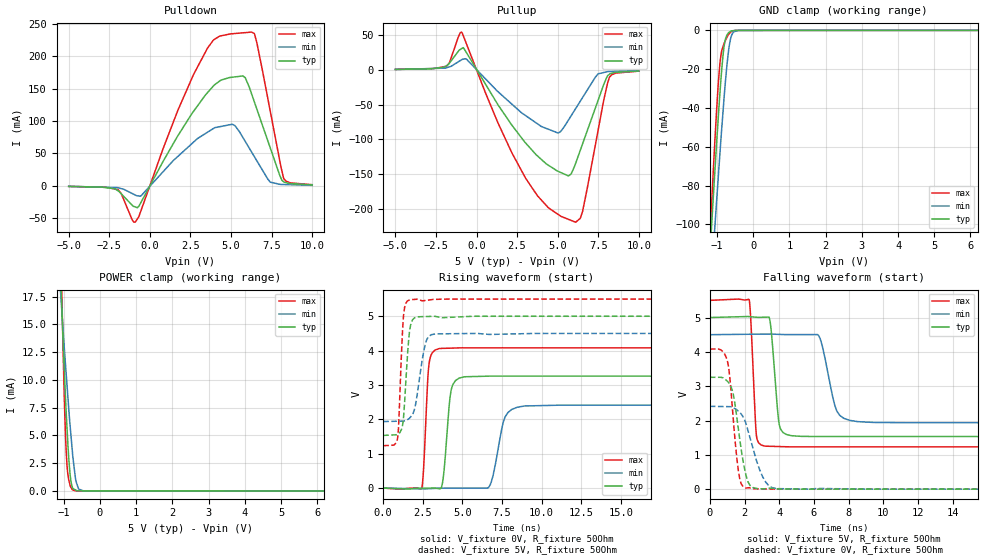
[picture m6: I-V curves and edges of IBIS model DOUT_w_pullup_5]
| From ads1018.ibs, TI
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|   DOUT Model 5 V model  Config Register bit3=0
[Model] DOUT_w_pullup_5
|  Signals  DOUT/_DRDY(9)
|   bit 3 of the Config Registor is zero
Model_type   3-state
Polarity   Non-Inverting
Enable   Active-Low
Vmeas = 2.5
Vref = 2.5
Cref = 15pF
Rref = 50|
|   typ   min   max
|   (nom PVT)   (Fast PVT)   (slow PVT)
C_comp   1.8834020e-12  1.5236910e-12  2.2665370e-12
|   typ   min   max
|   (nom PVT)   (slow PVT)   (Fast PVT)
|C_comp (ON state)   2.6065280e-12  2.2751560e-12  4.1907400e-12
|C_comp (OFF state)   2.4127670e-12  2.2979320e-12  3.1339800e-12
| Where   nom PVT is  Nominal Process, 5V, 27C
|   Fast PVT is Strong or Fast Process, 5.5V, -40C
|   Slow PVT is Weak or Slow Process, 4.5V, 125C
| variable   typ   min   max
[Voltage Range]   5   4.5   5.5
[Temperature Range]   27   125   -40
|Operating Temperature   27   125   -40
[Pullup Reference]   5   4.5   5.5
[Pulldown Reference]   0   0   0
[Power Clamp Reference]   5   4.5   5.5
[GND Clamp Reference]   0   0   0
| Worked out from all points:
|   slope of the pulldown table from 0 to 0.75 V, typ, clamps not added: 21.6 ohm
|   slope of the pullup table from 0 to 0.75 V, typ, clamps not added: 25.9 ohm
|   GND clamp passes 1 mA (typ) near -0.67 V on its own axis
|   POWER clamp passes 1 mA (typ) near -0.81 V on its own axis
|   falling waveform, V_fixture 5V, R_fixture 50Ohm: 20-80 % time 327ps typ, 636ps min, 228ps max; typ from 5 V to 1.53 V
|   rising waveform, V_fixture 0V, R_fixture 50Ohm: 20-80 % time 342ps typ, 600ps min, 247ps max; typ from 0 V to 3.26 V
|   rising waveform, V_fixture 5V, R_fixture 50Ohm: 20-80 % time 296ps typ, 513ps min, 232ps max; typ from 1.53 V to 5 V
|   falling waveform, V_fixture 0V, R_fixture 50Ohm: 20-80 % time 566ps typ, 869ps min, 426ps max; typ from 3.26 V to 0 V
[Pulldown]
|   Voltage   I(typ)   I(min)   I(max)
-5V       -725.3uA   -519.1uA   -702.5uA
-1.982V   -7.151mA   -2.659mA   -5.43mA
-904.6mV  -32.3mA    -13.94mA   -55.69mA
1.743V    78.08mA    45.97mA    117.7mA
3.543V    143.6mA    82.65mA    212mA
5.073V    167.5mA    95.02mA    234.4mA
5.878V    166.7mA    68.46mA    236.2mA
6.262V    142mA      52.38mA    237mA
6.588V    118.4mA    38.77mA    220.8mA
7.411V    58.87mA    5.98mA     115.6mA
8.232V    6.647mA    2.238mA    12.34mA
10V       1.629mA    964.4uA    1.981mA
[GND Clamp]
|   Voltage   I(typ)   I(min)   I(max)
-5V       -1.404A    -1.291A    -1.638A
-1.227V   -124.7mA   -148.3mA   -117.9mA
-1.165V   -105mA     -130.4mA   -94.43mA
-1.148V   -99.65mA   -125.6mA   -88.3mA
-1.058V   -71.83mA   -100.5mA   -56.01mA
-970.8mV  -46.2mA    -76.72mA   -28.63mA
-913.3mV  -30.33mA   -61.39mA   -15.69mA
-788.4mV  -6.224mA   -30.65mA   -6.039mA
-679.5mV  -1.158mA   -10.05mA   -2.032mA
-611.3mV  -337.6uA   -3.284mA   -608uA
-399.6mV  -32.58uA   -25.18uA   -58.78uA
10V       0A         0A         0A
[Pullup]
|   Voltage   I(typ)   I(min)   I(max)
-5V       576.2uA    454.8uA    606.3uA
-1.857V   5.713mA    2.967mA    5.127mA
-922.9mV  30.49mA    14.44mA    54.34mA
1.341V    -51.05mA   -31.91mA   -77.47mA
3.01V     -105.1mA   -65.73mA   -155.5mA
5.031V    -146.2mA   -91mA      -208.3mA
5.667V    -152.8mA   -72.14mA   -215.4mA
6.1V      -134.9mA   -56mA      -219.4mA
6.533V    -106.5mA   -39.85mA   -203.8mA
7.481V    -44.37mA   -5.99mA    -88.03mA
8.171V    -6.695mA   -2.423mA   -11.57mA
10V       -1.583mA   -1.032mA   -1.861mA
[POWER Clamp]
|   Voltage   I(typ)   I(min)   I(max)
-5V       476.7mA    315.9mA    750.7mA
-1.072V   18.22mA    17.1mA     20.63mA
-1.047V   15.95mA    15.84mA    16.68mA
-970.8mV  9.805mA    12.19mA    6.818mA
-944.3mV  7.828mA    11.02mA    4.358mA
-913.3mV  5.861mA    9.651mA    2.434mA
-825.6mV  1.5mA      5.9mA      505.4uA
-759.9mV  310.6uA    3.455mA    96.84uA
-660.1mV  66.56uA    835.5uA    9.12uA
-590.9mV  6.546uA    170.3uA    9.061uA
-456.8mV  6.463uA    5.004uA    8.946uA
10V       0A         0A         0A
[Ramp]
R_load = 50
|   typ   min   max
dV/dt_r   1.95497/3.39673e-010   1.44792/5.95804e-010   2.44883/2.46868e-010
dV/dt_f   2.08044/3.23153e-010   1.53815/6.31012e-010   2.56058/2.27292e-010
[Falling Waveform]
V_fixture = 5V
V_fixture_min = 4.5V
V_fixture_max = 5.5V
R_fixture = 50Ohm
C_fixture = 0F
|   Time   V(typ)   V(min)   V(max)
0s        5V         4.5V       5.5V
2.265ns   5.026V     4.512V     5.519V
2.681ns   5.009V     4.515V     1.582V
3.182ns   5.01V      4.517V     1.253V
4.008ns   1.869V     4.509V     1.241V
4.712ns   1.557V     4.503V     1.233V
6.273ns   1.534V     4.472V     1.233V
7.317ns   1.533V     2.281V     1.233V
8.521ns   1.533V     1.968V     1.233V
50ns      1.533V     1.936V     1.232V
[Rising Waveform]
V_fixture = 0V
V_fixture_min = 0V
V_fixture_max = 0V
R_fixture = 50Ohm
C_fixture = 0F
|   Time   V(typ)   V(min)   V(max)
0s        829.1pV    1.313nV    740.3pV
2.423ns   -1.466mV   -20.94mV   -12.68mV
2.893ns   -445.1uV   -17.73mV   3.606V
3.555ns   -19.94mV   -1.51mV    4.062V
4.296ns   2.857V     -1.295mV   4.072V
5.126ns   3.238V     -1.053mV   4.081V
6.684ns   3.257V     37.03mV    4.081V
7.689ns   3.258V     2.062V     4.081V
8.914ns   3.258V     2.389V     4.081V
50ns      3.258V     2.413V     4.081V
[Rising Waveform]
V_fixture = 5V
V_fixture_min = 4.5V
V_fixture_max = 5.5V
R_fixture = 50Ohm
C_fixture = 0F
|   Time   V(typ)   V(min)   V(max)
0s        1.533V     1.936V     1.232V
906.7ps   1.563V     1.946V     1.44V
981.2ps   1.589V     1.947V     1.887V
1.289ns   2.089V     1.95V      5.037V
1.548ns   3.958V     1.996V     5.45V
1.72ns    4.713V     2.063V     5.481V
2.049ns   4.965V     2.443V     5.492V
2.69ns    4.991V     4.241V     5.461V
3.279ns   4.998V     4.486V     5.491V
50ns      5V         4.5V       5.5V
[Falling Waveform]
|Gnd
V_fixture = 0V
V_fixture_min = 0V
V_fixture_max = 0V
R_fixture = 50Ohm
C_fixture = 0F
|   Time   V(typ)   V(min)   V(max)
0s        3.258V     2.413V     4.081V
1.015ns   3.144V     2.404V     3.728V
1.145ns   3.055V     2.403V     3.293V
1.33ns    2.816V     2.373V     2.173V
1.647ns   1.747V     2.268V     528.8mV
2.077ns   418.6mV    1.924V     32.49mV
2.319ns   105.6mV    1.492V     36.06mV
3.037ns   8.508mV    369mV      8.224mV
3.9ns     10.23mV    16.15mV    286.2uV
50ns      829.1pV    1.313nV    740.3pV
